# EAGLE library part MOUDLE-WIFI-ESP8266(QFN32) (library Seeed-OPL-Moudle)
113990084
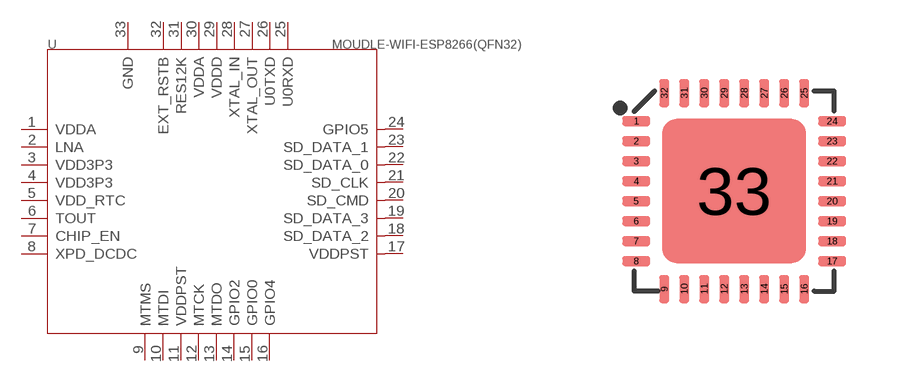
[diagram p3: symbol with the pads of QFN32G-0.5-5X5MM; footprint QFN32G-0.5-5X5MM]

Designator prefix U

## MOUDLE-WIFI-ESP8266(QFN32) (MPN: ESP8266-04; VALUE: ESP8266-Small)  [QFN32G-0.5-5X5MM]
1  VDDA
2  LNA
3  VDD3P3
4  VDD3P3
5  VDD_RTC
6  TOUT
7  CHIP_EN
8  XPD_DCDC
9  MTMS
10  MTDI
11  VDDPST
12  MTCK
13  MTDO
14  GPIO2
15  GPIO0
16  GPIO4
17  VDDPST
18  SD_DATA_2
19  SD_DATA_3
20  SD_CMD
21  SD_CLK
22  SD_DATA_0
23  SD_DATA_1
24  GPIO5
25  U0RXD
26  U0TXD
27  XTAL_OUT
28  XTAL_IN
29  VDDD
30  VDDA
31  RES12K
32  EXT_RSTB
33  GND

## Footprint QFN32G-0.5-5X5MM (pad centres in mm)
smd 0.7 x 0.25: 1 -2.45,1.75; 2 -2.45,1.25; 3 -2.45,0.75; 4 -2.45,0.25; 5 -2.45,-0.25; 6 -2.45,-0.75; 7 -2.45,-1.25; 8 -2.45,-1.75; 17 2.45,-1.75; 18 2.45,-1.25; 19 2.45,-0.75; 20 2.45,-0.25; 21 2.45,0.25; 22 2.45,0.75; 23 2.45,1.25; 24 2.45,1.75
smd 0.25 x 0.7: 9 -1.75,-2.45; 10 -1.25,-2.45; 11 -0.75,-2.45; 12 -0.25,-2.45; 13 0.25,-2.45; 14 0.75,-2.45; 15 1.25,-2.45; 16 1.75,-2.45; 25 1.75,2.45; 26 1.25,2.45; 27 0.75,2.45; 28 0.25,2.45; 29 -0.25,2.45; 30 -0.75,2.45; 31 -1.25,2.45; 32 -1.75,2.45
smd 3.6 x 3.6: 33 0,0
